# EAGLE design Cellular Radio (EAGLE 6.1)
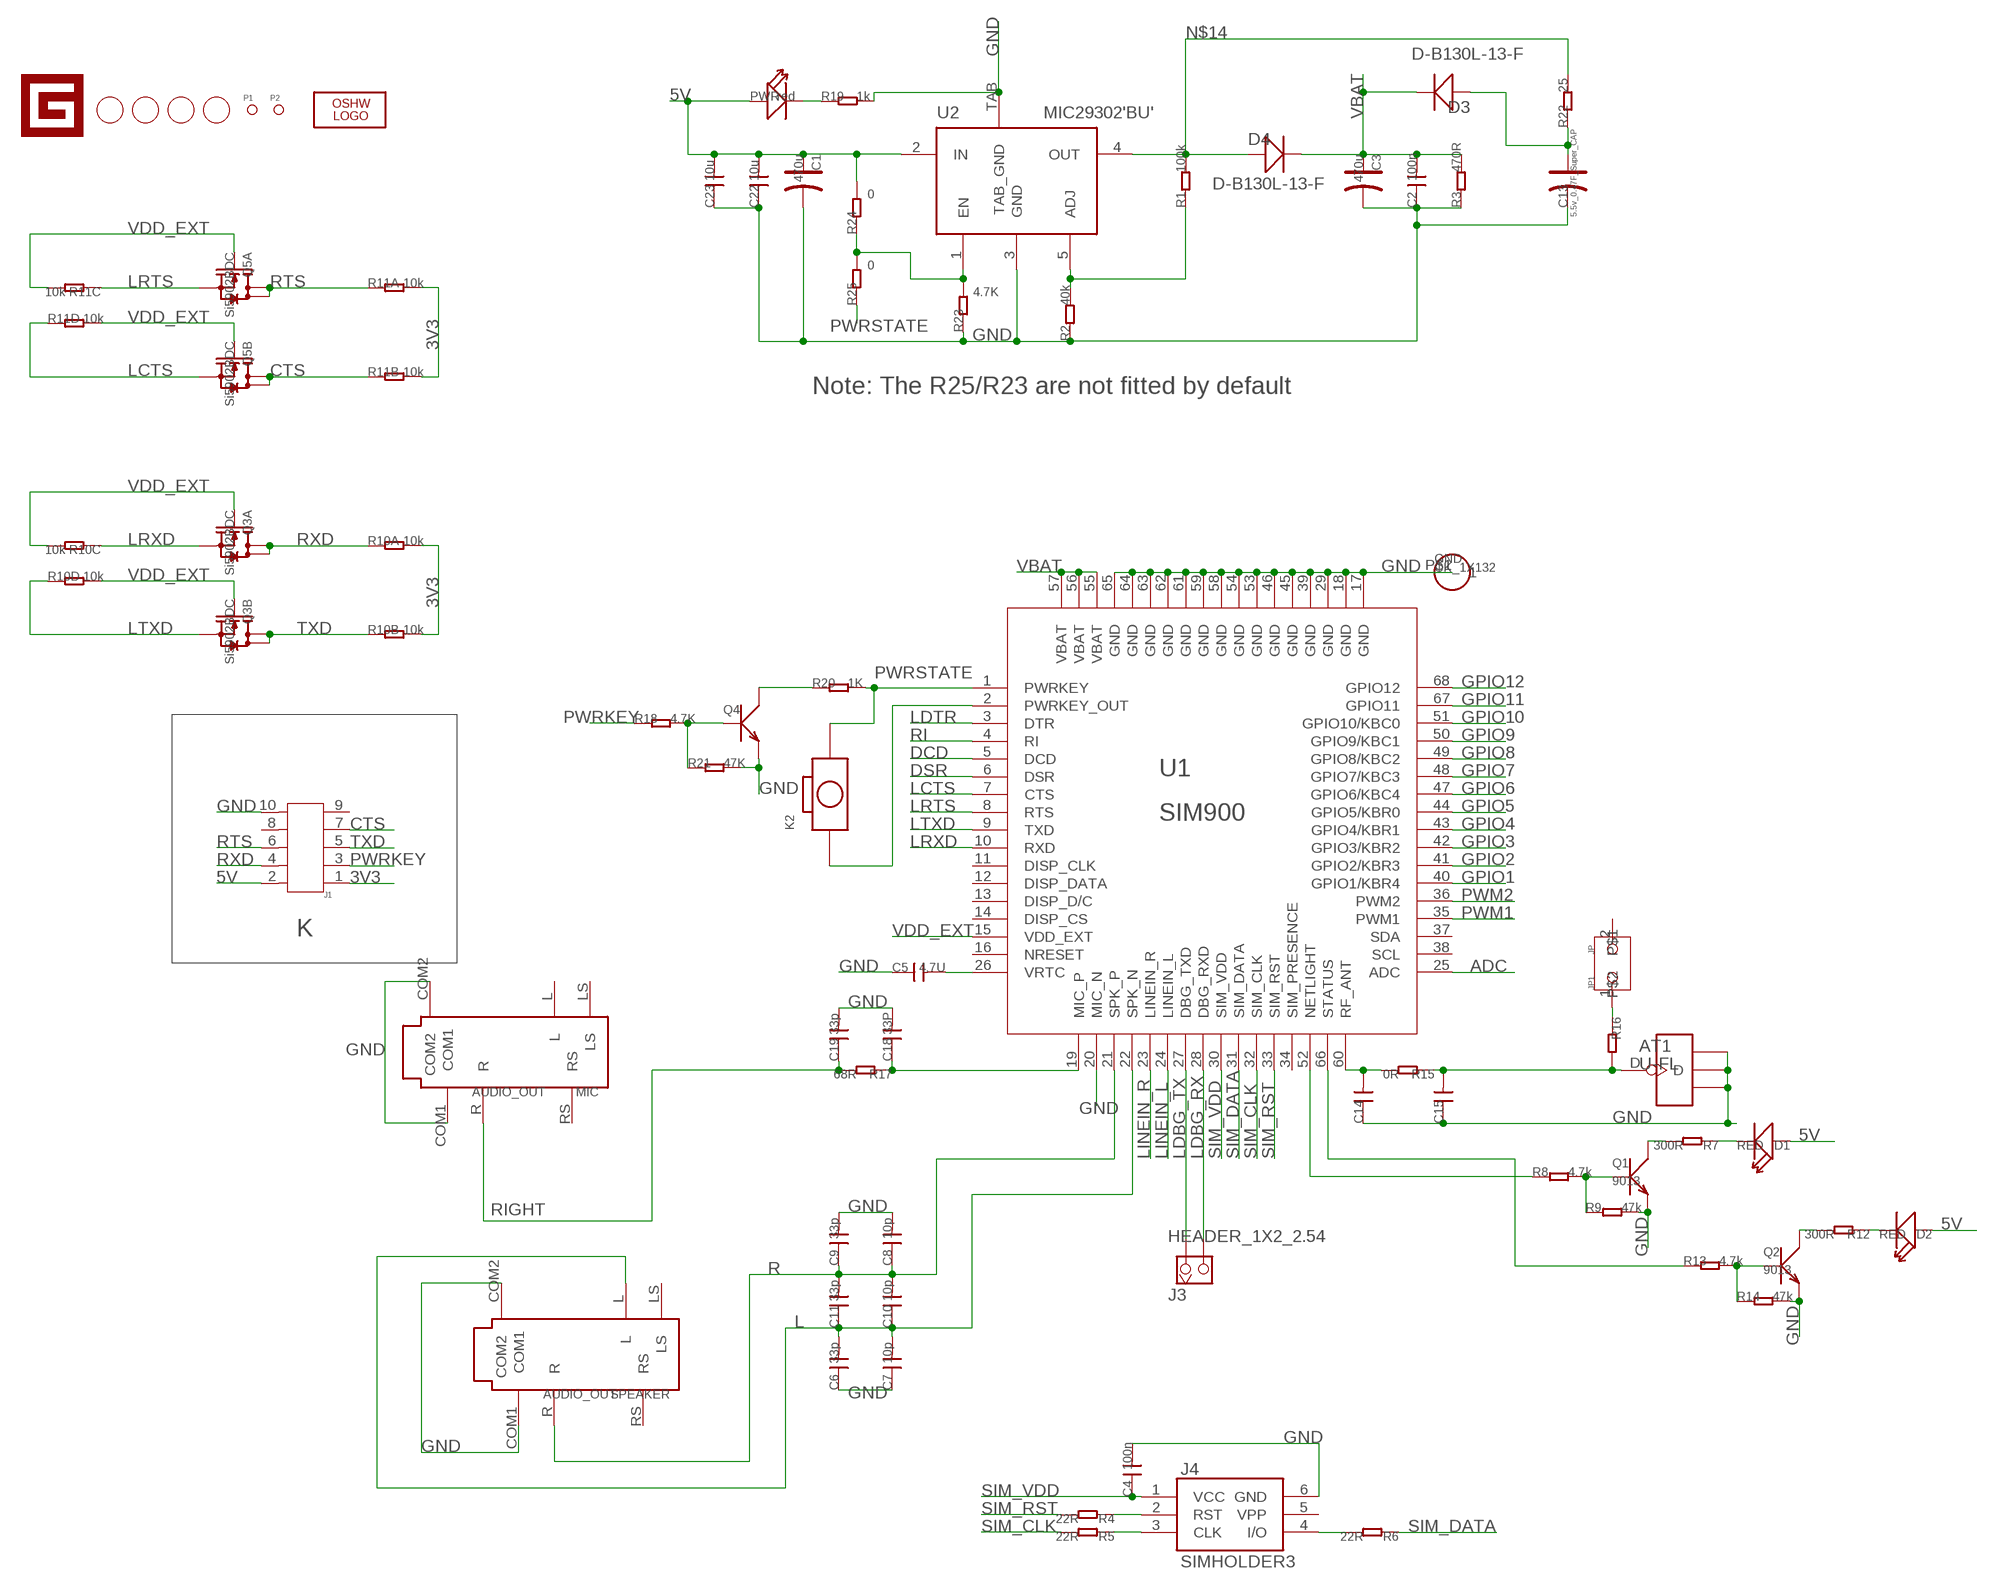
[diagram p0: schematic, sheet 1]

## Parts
AT1  U-FL  [U-FL]
C1  470u  006-CAP_AVX_D  [AVX_D]
C2  100n  006-C0805  [0805@1]
C3  470u  006-CAP_AVX_D  [AVX_D]
C4  100n  006-C0603  [0603@1]
C5  4.7U  006-C0805  [0805@1]
C6  33p  006-C0402  [0402]
C7  10p  006-C0402  [0402]
C8  10p  006-C0402  [0402]
C9  33p  006-C0402  [0402]
C10  10p  006-C0402  [0402]
C11  33p  006-C0402  [0402]
C13  5.5v_0.47F_Super_CAP  006-CAP_UC13  [SUPER_CAP_R13]
C14  006-C0402  [0402]
C15  006-C0402  [0402]
C18  33P  006-C0603  [0603@1]
C19  33p  006-C0603  [0603@1]
C22  10u  006-C0805  [0805@1]
C23  10u  006-C0805  [0805@1]
D1  RED  007-LED0603  [D0603]
D2  RED  007-LED0603  [D0603]
D3  D-B130L-13-F  [SMA]
D4  D-B130L-13-F  [SMA]
GND  CK_1X132  [CK_1X1]
J1  HEADER-SHF-105-01-L-D-SM  [SHF-105-01-L-D-SM]
J3  HEADER_1X2_2.54  [CK_1*2]
J4  SIMHOLDER3  [SIMHOLDER3]
JP1  JP  [JP]
K2  BOTTON_1_DP  [BTN_5.0_RST]
LOGO1  LOGO-OSHW-FILLX0150-NT  [OSHW_FILLX150_NOTEXT]
MIC  AUDIO_OUT  AUDIO  [3.5MM_AUDIO]
P1  PAD-MARK  [ROUND-MARK-0.635]
P2  PAD-MARK  [ROUND-MARK-0.635]
PWR  red  007-LED0603  [D0603]
Q1  9013  010-NPNSOT23  [SOT23]
Q2  9013  010-NPNSOT23  [SOT23]
Q3  Si5902BDC  010-DUAL-N-MOSFET_1206-8  [1206-8]
Q4  TRANSISTOR-NPN-SOT23''  [SOT23]
Q5  Si5902BDC  010-DUAL-N-MOSFET_1206-8  [1206-8]
R1  100k  005-R0805  [0805@1]
R2  40k  005-R0805  [0805@1]
R3  470R  005-R0805  [0805@1]
R4  22R  005-R0603  [0603@1]
R5  22R  005-R0603  [0603@1]
R6  22R  005-R0603  [0603@1]
R7  300R  005-R0603  [0603@1]
R8  4.7k  005-R0603  [0603@1]
R9  47k  005-R0603  [0603@1]
R10  10k  005-4R_1206  [R1206-8]
R11  10k  005-4R_1206  [R1206-8]
R12  300R  005-R0603  [0603@1]
R13  4.7k  005-R0603  [0603@1]
R14  47k  005-R0603  [0603@1]
R15  0R  005-R0402  [0402]
R16  005-R0402  [0402]
R17  68R  005-R0603  [0603@1]
R18  4.7K  005-R0402  [0402]
R19  1k  005-R0603  [0603@1]
R20  1K  005-R0402  [0402]
R21  47K  005-R0402  [0402]
R22  25  R-0603  [0603]
R23  4.7K  R-0603  [0603]
R24  0  R-0603  [0603]
R25  0  R-0603  [0603]
SPEAKER  AUDIO_OUT  AUDIO  [3.5MM_AUDIO]
U1  SIM900  [SIM900]
U2  MIC29302'BU'  [TO-263]
U$1  LOGO-GADGETEER-NORMAL  [GADGETEER-SILK]
U$2  PAD-HOLE'3.2/7.0'  [HOLE-D-3.2/7.0]
U$3  PAD-HOLE'3.2/7.0'  [HOLE-D-3.2/7.0]
U$4  PAD-HOLE'3.2/7.0'  [HOLE-D-3.2/7.0]
U$5  PAD-HOLE'3.2/7.0'  [HOLE-D-3.2/7.0]

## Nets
3V3: J1.1 R10.7 R10.8 R11.7 R11.8
5V: C1.+ C22.2 C23.2 D1.+ D2.+ J1.2 PWR.+ R24.2 U2.2(IN)
ADC: U1.25(ADC)
CTS: J1.7 Q5.5(B:D) Q5.6(B:D) R11.2
DCD: U1.5(DCD)
DSR: U1.6(DSR)
GND: AT1.GND1 AT1.GND2 AT1.GND3 C1.- C2.1 C3.- C4.2 C5.1 C6.1 C7.1 C8.2 C9.2 C13.- C14.1 C15.1 C18.2 C19.2 C22.1 C23.1 GND.P$1 J1.10 J4.6(GND) MIC.COM1 MIC.COM2 Q1.2(E) Q2.2(E) Q4.2(E) R2.1 R3.1 R9.2 R14.2 R19.2 R21.2 R23.1 SPEAKER.COM1 SPEAKER.COM2 U1.17(GND) U1.18(GND) U1.20(MIC_N) U1.29(GND) U1.39(GND) U1.45(GND) U1.46(GND) U1.53(GND) U1.54(GND) U1.58(GND) U1.59(GND) U1.61(GND) U1.62(GND) U1.63(GND) U1.64(GND) U1.65(GND) U2.3(GND) U2.TAB(TAB_GND)
GPIO1: U1.40(GPIO1/KBR4)
GPIO2: U1.41(GPIO2/KBR3)
GPIO3: U1.42(GPIO3/KBR2)
GPIO4: U1.43(GPIO4/KBR1)
GPIO5: U1.44(GPIO5/KBR0)
GPIO6: U1.47(GPIO6/KBC4)
GPIO7: U1.48(GPIO7/KBC3)
GPIO8: U1.49(GPIO8/KBC2)
GPIO9: U1.50(GPIO9/KBC1)
GPIO10: U1.51(GPIO10/KBC0)
GPIO11: U1.67(GPIO11)
GPIO12: U1.68(GPIO12)
L: C6.2 C7.2 C10.1 C11.1 SPEAKER.L U1.22(SPK_N)
LCTS: Q5.3(B:S) R11.4 U1.7(CTS)
LDBG_RX: J3.2 U1.28(DBG_RXD)
LDBG_TX: J3.1 U1.27(DBG_TXD)
LDTR: U1.3(DTR)
LINEIN_L: U1.24(LINEIN_L)
LINEIN_R: U1.23(LINEIN_R)
LRTS: Q5.1(A:S) R11.3 U1.8(RTS)
LRXD: Q3.1(A:S) R10.3 U1.10(RXD)
LTXD: Q3.3(B:S) R10.4 U1.9(TXD)
N$1: C14.2 R15.2 U1.60(RF_ANT)
N$2: R1.1 R2.2 U2.5(ADJ)
N$3: Q1.3(C) R7.2
N$4: J4.4(I/O) R6.2
N$5: J4.3(CLK) R5.1
N$6: J4.2(RST) R4.1
N$7: D1.- R7.1
N$8: Q1.1(B) R8.2 R9.1
N$9: Q4.3(C) R20.1
N$10: R8.1 U1.52(NETLIGHT)
N$11: Q4.1(B) R18.2 R21.1
N$12: C5.2 U1.26(VRTC)
N$13: C18.1 R17.1 U1.19(MIC_P)
N$14: D4.P$2(+) R1.2 R22.2 U2.4(OUT)
N$15: C13.+ D3.P$2(+) R22.1
N$16: Q2.3(C) R12.2
N$17: D2.- R12.1
N$18: Q2.1(B) R13.2 R14.1
N$19: R23.2 R24.1 R25.2 U2.1(EN)
N$20: R13.1 U1.66(STATUS)
N$21: AT1.D C15.2 R15.1 R16.2
N$22: JP1.1 R16.1
N$24: K2.P$1 U1.2(PWRKEY_OUT)
N$53: PWR.- R19.1
PWM1: U1.35(PWM1)
PWM2: U1.36(PWM2)
PWRKEY: J1.3 R18.1
PWRSTATE: K2.P$2 R20.2 R25.1 U1.1(PWRKEY)
R: C8.1 C9.1 C10.2 C11.2 SPEAKER.R U1.21(SPK_P)
RI: U1.4(RI)
RIGHT: C19.1 MIC.R R17.2
RTS: J1.6 Q5.7(A:D) Q5.8(A:D) R11.1
RXD: J1.4 Q3.7(A:D) Q3.8(A:D) R10.1
SIM_CLK: R5.2 U1.32(SIM_CLK)
SIM_DATA: R6.1 U1.31(SIM_DATA)
SIM_RST: R4.2 U1.33(SIM_RST)
SIM_VDD: C4.1 J4.1(VCC) U1.30(SIM_VDD)
TXD: J1.5 Q3.5(B:D) Q3.6(B:D) R10.2
VBAT: C2.2 C3.+ D3.P$1(-) D4.P$1(-) R3.2 U1.55(VBAT) U1.56(VBAT) U1.57(VBAT)
VDD_EXT: Q3.2(A:G) Q3.4(B:G) Q5.2(A:G) Q5.4(B:G) R10.5 R10.6 R11.5 R11.6 U1.15(VDD_EXT)
Unconnected: J1.8 J1.9 J4.5(VPP) JP1.2 MIC.L MIC.LS MIC.RS SPEAKER.LS SPEAKER.RS U1.11(DISP_CLK) U1.12(DISP_DATA) U1.13(DISP_D/C) U1.14(DISP_CS) U1.16(NRESET) U1.34(SIM_PRESENCE) U1.37(SDA) U1.38(SCL)

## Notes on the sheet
- Note: The R25/R23 are not fitted by default
- K

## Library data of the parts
AT1 = CPT_SMD:U-FL
C1 C3 C13 = Discrete:006-CAP*: Electrolytic Capacitors,Tantalum Capacitors and Super Capacitors
C2 C4-C11 C14 C15 C18 C19 C22 C23 = Discrete:006-C*: Ceramic Capacitors
D1 D2 PWR = Discrete:007-LED*
D3 D4 = Discrete:D*
GND = CONNECTER:CK_1X1
J1 = Connector:HEADER-SHF-105-01-L-D-SM
J3 = CONNECTER:HEADER_1X2
J4 = SparkFun2:SIMHOLDER3
JP1 = mySeeed:JP
K2 = CPT_SMD:BOTTON_1
LOGO1 = Logo:LOGO-OSHW-FILL
MIC SPEAKER = MusicShield:AUDIO
P1 P2 = Discreter:PAD-MARK
Q1 Q2 = Discrete:010-NPN*: NPN audion
Q3 Q5 = Discrete:010-DUAL-N-MOSFET*: Si5902BDC Si5904DC Si5908DC Si5920DC
Q4 = Discreter:TRANSISTOR-NPN*: NPN audion
R1-R9 R12-R21 = Discrete:005-R*
R10 R11 = Discrete:005-4R*: Resistor Array
R22-R25 = Discrete:R*
U1 = ICs_v54:SIM900
U2 = ICs_v54:MIC29302
U$1 = Logo:LOGO-GADGETEER
U$2-U$5 = Discreter:PAD-HOLE

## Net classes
0 default: width 0.203 mm, drill 0.305 mm, clearance 0.152 mm

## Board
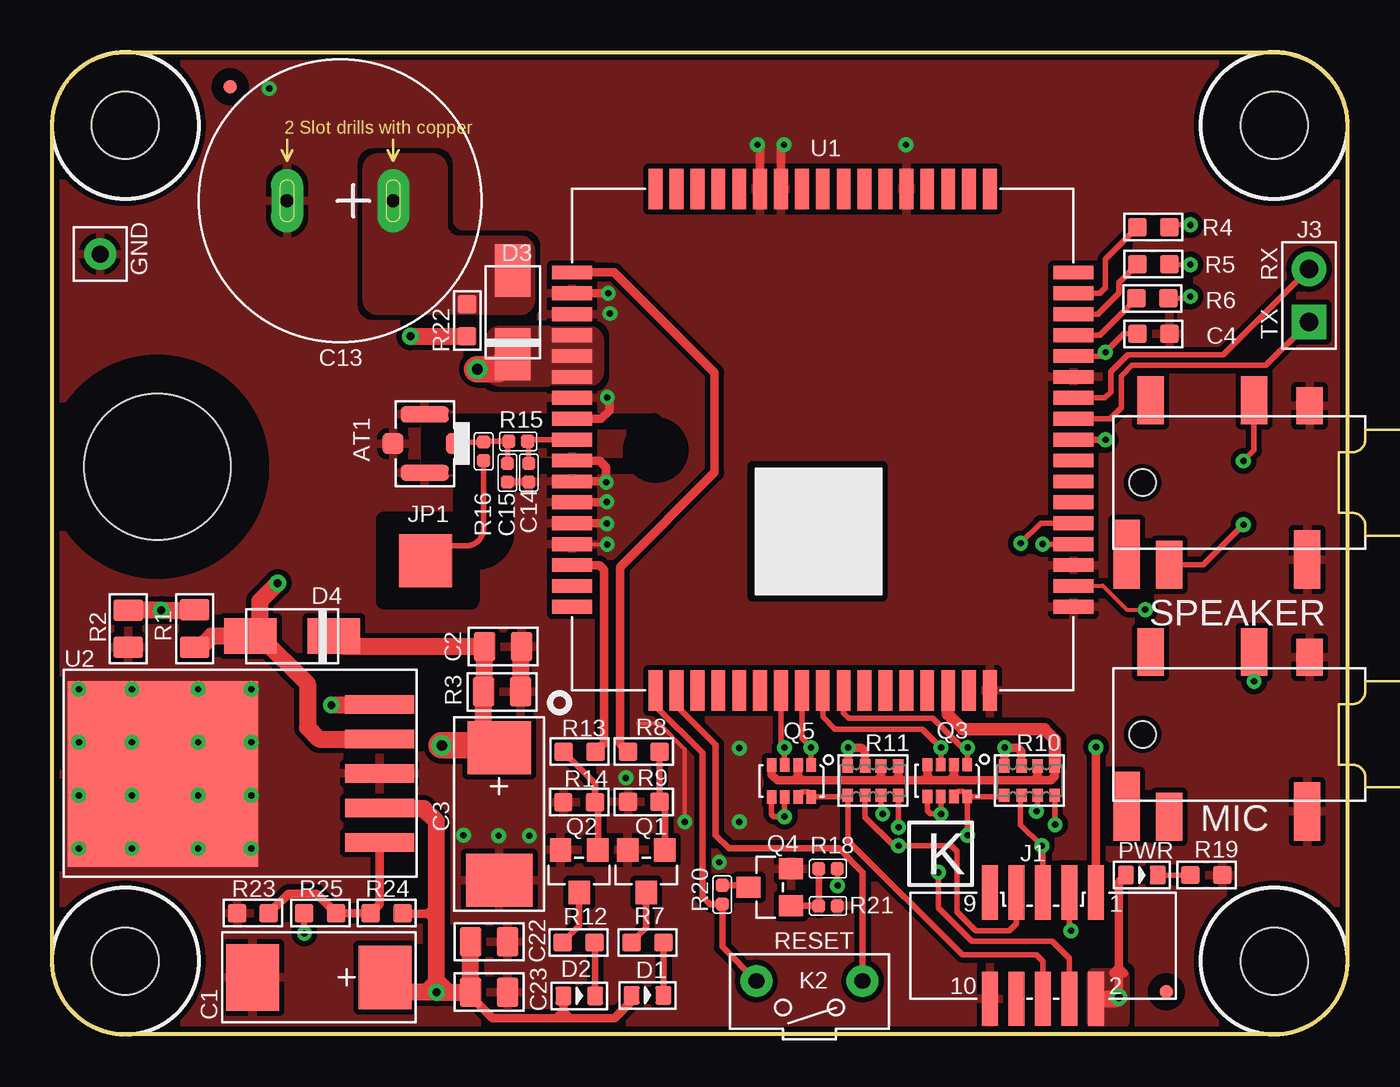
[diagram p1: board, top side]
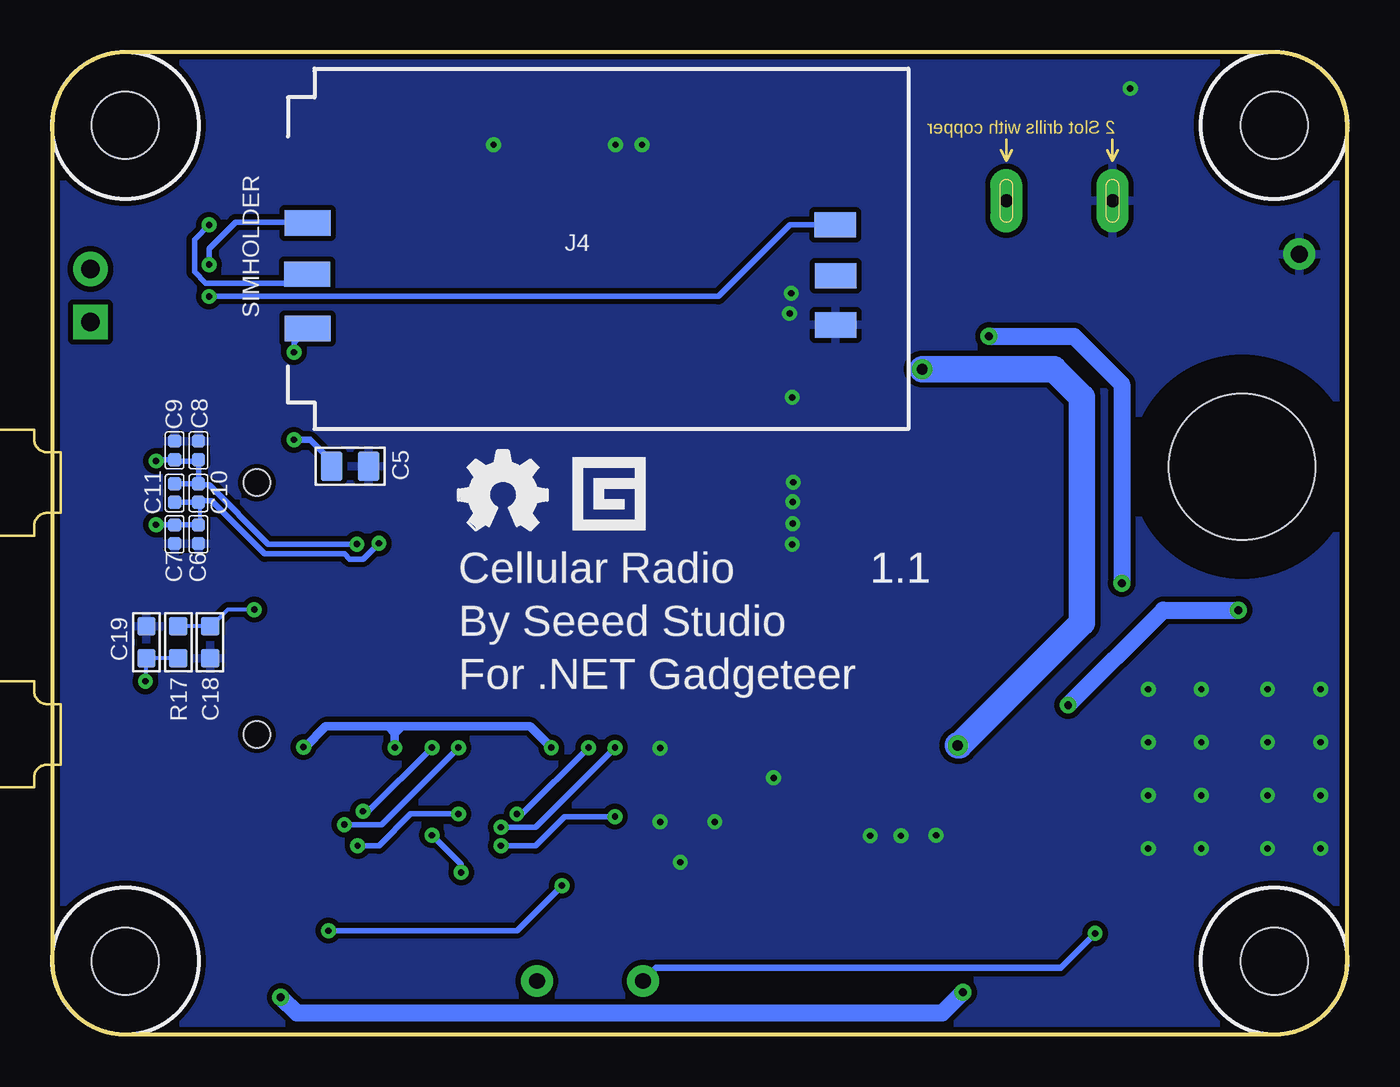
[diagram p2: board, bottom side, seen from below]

Size 62 x 47 mm. Coordinates in mm from the lower left corner, seen from the top.
Outline: 62,3.5 arc-90 58.5,0 3.5,0 arc-90 0,3.5 0,43.5 arc-90 3.5,47 58.5,47 arc-90 62,43.5 62,3.5
Copper layers (1*16): Top 0.035mm / dielectric 1.5mm / Bottom 0.035mm
Design rules: minimum track width 8mil, minimum drill 12mil, track to track 6mil, track to pad 6mil, pad to pad 6mil, via to via 6mil, smd to smd 6mil, copper to edge 10mil, drill to drill 8mil, minimum pad ring 10mil, minimum via ring 8mil, stop-mask expansion 4mil, vias tented up to drill 100mil, thermal gap 10mil
Holes 7 mm at 5.04,27.16
tRestrict: area 0,22.2 to 10,32.2; area 24.1,34.8 to 25.5,35.2; area 24.3,29.7 to 25.7,30.1; area 24.1,23.8 to 25.5,24.1; area 24.1,25.8 to 25.5,26.2; area 24.1,24.8 to 25.5,25.2; area 34.2,39.8 to 34.5,41.2; area 33.5,21 to 39.8,27.2; 14 lines
bRestrict: area 0,22.2 to 10,32.2

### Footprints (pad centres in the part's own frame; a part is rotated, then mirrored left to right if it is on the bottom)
U-FL = smd 1.016 x 1.016: D -1.524,0; GND3 1.524,0 | smd 2.286 x 0.762: GND1 0,1.397; GND2 0,-1.397
AVX_D = smd 2.54 x 3.048: + -3.175,0 | smd 2.54 x 3.175: - 3.175,0
0805@1 = smd 1.016 x 1.397: 1 -0.889,0; 2 0.889,0
0603@1 = smd 0.889 x 0.889: 1 -0.762,0; 2 0.762,0
0402 = smd 0.635 x 0.635: 1 -0.445,0; 2 0.445,0
SUPER_CAP_R13 = drill 0.635 pad 1.524 long: + -2.54,0; - 2.54,0
D0603 = smd 0.762 x 0.889: + -0.762,0; - 0.762,0
SMA = smd 2.5 x 1.7: P$1 -2,0; P$2 2,0
CK_1X1 = drill 0.813 pad 1.524: P$1 0,0
SHF-105-01-L-D-SM = smd 0.762 x 2.6: 1 -2.54,-2.54; 2 -2.54,2.54; 3 -1.27,-2.54; 4 -1.27,2.54; 5 0,-2.54; 6 0,2.54; 7 1.27,-2.54; 8 1.27,2.54; 9 2.54,-2.546; 10 2.54,2.54
CK_1*2 = drill 0.889 pad 1.651 square: 1 0,1.27 | drill 0.889 pad 1.651: 2 0,-1.27
SIMHOLDER3 = smd 2.2 x 1.2: 1 0.95,4.81; 2 0.91,7.41; 3 0.95,9.86 | smd 2 x 1.2: 4 26.2,9.78; 5 26.22,7.34; 6 26.22,4.98
JP = smd 1.27 x 2.54: 1 -0.635,0; 2 0.635,0
BTN_5.0_RST = drill 0.762 pad 1.524: P$1 0,2.54; P$2 0,-2.54
3.5MM_AUDIO = smd 1.27 x 1.778: COM1 -4.572,3.683 | smd 1.27 x 2.794: COM2 -4.699,-3.683 | smd 1.27 x 2.286: L -11.303,-3.937; R -7.239,3.937; RS -12.192,3.937 | smd 1.27 x 3.302: LS -13.335,-3.429 | hole 1.27: -12.573,0
ROUND-MARK-0.635 = smd 0.635 x 0.635: P$1 0,0
SOT23@1 = smd 1.016 x 1.143: 1 -0.889,-1.016; 2 0.889,-1.016; 3 0,1.016
1206-8 = smd 0.457 x 0.635: 1 -0.953,-0.762; 2 -0.318,-0.762; 3 0.318,-0.762; 4 0.953,-0.762; 5 0.953,0.762; 6 0.318,0.762; 7 -0.318,0.762; 8 -0.953,0.762
SOT23 = smd 1.016 x 1.143: 1 -0.889,-1.016; 2 0.889,-1.016; 3 0,1.016
R1206-8 = smd 0.508 x 0.635: 1 -1.206,-0.699; 2 -0.381,-0.699; 3 0.381,-0.699; 4 1.206,-0.699; 5 1.206,0.699; 6 0.381,0.699; 7 -0.381,0.699; 8 -1.206,0.699
0603 = smd 0.889 x 0.889: 1 -0.762,0; 2 0.762,0
SIM900 = smd 1.93 x 0.66: 1 -12,8; 2 -12,7; 3 -12,6; 4 -12,5; 5 -12,4; 6 -12,3; 7 -12,2; 8 -12,1; 9 -12,0; 10 -12,-1; 11 -12,-2; 12 -12,-3; 13 -12,-4; 14 -12,-5; 15 -12,-6; 16 -12,-7; 17 -12,-8; 35 12,-8; 36 12,-7; 37 12,-6; 38 12,-5; 39 12,-4; 40 12,-3; 41 12,-2; 42 12,-1; 43 12,0; 44 12,1; 45 12,2; 46 12,3; 47 12,4; 48 12,5; 49 12,6; 50 12,7; 51 12,8 | smd 0.66 x 1.93: 18 -8,-12; 19 -7,-12; 20 -6,-12; 21 -5,-12; 22 -4,-12; 23 -3,-12; 24 -2,-12; 25 -1,-12; 26 0,-12; 27 1,-12; 28 2,-12; 29 3,-12; 30 4,-12; 31 5,-12; 32 6,-12; 33 7,-12; 34 8,-12; 52 8,12; 53 7,12; 54 6,12; 55 5,12; 56 4,12; 57 3,12; 58 2,12; 59 1,12; 60 0,12; 61 -1,12; 62 -2,12; 63 -3,12; 64 -4,12; 65 -5,12; 66 -6,12; 67 -7,12; 68 -8,12
TO-263 = smd 3.302 x 0.889: 1 3.302,-3.302; 2 3.302,-1.651; 3 3.302,0; 4 3.302,1.651; 5 3.302,3.302 | smd 9.12 x 8.89: TAB -7.071,-0.03
HOLE-D-3.2/7.0 = hole 3.2: 0,0

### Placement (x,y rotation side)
AT1  17.83,28.27 180 top
C1  12.76,2.73 180 top
C2  21.59,18.56 180 top
C3  21.4,10.54 270 top
C4  52.72,33.53 0 top
C5  47.74,27.19 180 bottom
C6  55,23.93 90 bottom
C7  56.14,23.93 90 bottom
C8  55,27.95 90 bottom
C9  56.14,27.95 90 bottom
C10  55,25.91 90 bottom
C11  56.14,25.91 90 bottom
C13  13.78,39.89 180 top
C14  22.81,26.88 90 top
C15  21.8,26.88 90 top
C18  54.44,18.76 270 bottom
C19  57.49,18.76 90 bottom
C22  20.92,4.44 180 top
C23  20.92,2.02 180 top
D1  28.5,1.86 0 top
D2  25.23,1.84 0 top
D3  22.05,34.55 90 top
D4  11.49,19.05 180 top
GND  2.29,37.34 0 top
J1  47.43,4.24 180 top
J3  60.17,35.36 180 top
J4  50.71,28.97 0 bottom
JP1  17.87,22.66 270 top
K2  36.25,2.55 270 top
LOGO1  42.55,24.14 0 bottom
MIC  64.78,14.36 0 top
P1  8.51,45.34 0 top
P2  53.34,2.04 0 top
PWR  52.16,7.62 0 top
Q1  9013  [SOT23@1]  28.44,7.81 180 top
Q2  9013  [SOT23@1]  25.23,7.81 180 top
Q3  42.85,12.14 180 top
Q4  34.35,7.04 90 top
Q5  35.39,12.12 180 top
R1  6.82,19.42 270 top
R2  3.64,19.41 90 top
R3  21.54,16.39 180 top
R4  52.72,38.63 180 top
R5  52.72,36.86 180 top
R6  52.67,35.22 0 top
R7  28.5,4.4 180 top
R8  28.32,13.53 0 top
R9  28.32,11.13 180 top
R10  46.79,12.14 0 top
R11  39.3,12.14 0 top
R12  25.2,4.4 180 top
R13  25.25,13.53 180 top
R14  25.23,11.11 180 top
R15  22.31,28.38 0 top
R16  20.65,27.9 90 top
R17  55.97,18.76 270 bottom
R18  37.14,7.93 180 top
R19  55.26,7.62 0 top
R20  32.08,6.69 270 top
R21  37.14,6.15 0 top
R22  19.87,34.17 270 top
R23  9.61,5.8 0 top
R24  16.01,5.8 0 top
R25  12.83,5.8 0 top
SPEAKER  64.78,26.41 0 top
U1  36.89,28.46 90 top
U2  12.37,12.49 0 top
U$1  34.93,26.29 0 bottom
U$2  3.5,3.5 0 top
U$3  3.5,43.5 0 top
U$4  58.5,43.5 0 top
U$5  58.5,3.5 0 top

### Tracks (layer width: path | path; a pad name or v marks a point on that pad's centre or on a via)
3V3  (via drill 0.3 pad 0.64)
  Top 0.406: R11.8 38.09,13.7 v38.11,13.72 38.74,13.72 38.91,13.55 R11.7 | R10.8 45.58,13.7 v45.6,13.72 46.23,13.72 46.41,13.55 R10.7 | J1.1 v49.97,13.74 v49.97,13.75
  Bottom 0.406: v38.11,13.72 39.12,14.74 45.27,14.74 | 45.6,14.74 45.93,14.74 | v49.97,13.75 49.89,13.75 48.9,14.74 45.93,14.74 | 45.6,14.41 45.6,14.74 | v45.6,13.72 45.6,14.25 45.6,14.41 | 45.27,14.74 45.6,14.41 | 45.27,14.74 45.6,14.74 | 45.6,14.41 45.93,14.74
5V  (via drill 0.38 pad 0.81)
  Top 0.254: 17.96,5.8 17.96,5.77
  Top 0.305: 27.74,1.7 D1.+
  Top 0.406: 27.74,1.7 27.74,1.58 26.93,0.77 24.77,0.77 | 24.14,0.77 24.39,0.77 | 24.39,0.77 24.77,0.77 | 24.47,1.07 24.47,0.85 24.39,0.77 | 24.47,1.1 D2.+ | 24.14,0.77 24.47,1.1 | 24.47,1.1 24.47,1.07 | 24.47,1.07 24.77,0.77 | 24.14,0.77 21.09,0.77 20.08,1.77 20.08,1.97 | 18.39,5.85 18.34,5.8 17.96,5.8 18.42,5.34 | 18.42,6.23 17.96,5.77 16.79,5.77 R24.2 | 16.52,10.8 15.67,10.8 U2.2 | v51.06,1.78 51.06,3.18 | 51.06,3.18 51.06,7.28 PWR.+ | 51.06,3.18 50.8,2.93 | 51.06,3.18 51.31,2.93
  Top 0.813: J1.2 50.98,1.7 v51.06,1.78 | 15.71,10.8 16.52,10.8 17.79,10.8 18.39,10.19 18.39,5.85 18.39,2.7 | v18.39,2.01 C23.2 | 18.42,2.55 18.4,2.57 18.4,2.69 18.39,2.7 | 18.42,2.55 18.93,2.04 | 18.42,2.55 17.89,2.02 | v18.39,2.01 16.65,2.01 C1.+ | v18.39,2.01 18.39,2.7 | C23.2 C22.2 | C23.2 arc-60 20.08,1.97
  Bottom 0.813: v51.06,1.78 50.3,1.02 19.38,1.02 v18.39,2.01
  pour Top (isolate 0.254, no thermals): 51.44,0.64 arc-90 51.19,0.39 49.92,0.39 arc-90 49.66,0.64 49.66,2.8 arc-90 49.92,3.05 51.19,3.05 arc-90 51.44,2.8
CTS  (via drill 0.3 pad 0.64)
  Top 0.254: Q5.6 35.06,11.35 v35.06,10.42 34.55,10.42 34.44,10.53 Q5.5 | J1.7 46.16,5.3 45.82,4.96 44.23,4.96 43.31,5.87 43.31,8.77 43.06,9.02 v40.52,9.02 40.29,9.02 38.91,10.4 R11.2
  Bottom 0.254: v35.06,10.42 37.47,10.42 38.87,9.02 v40.52,9.02
GND  (via drill 0.3 pad 0.64)
  Top 0.203: v30.28,10.16 30.28,13.64 29.06,14.86 28.05,14.86 | U1.65 v26.56,23.46 v26.57,23.45
  Top 0.305: C15.1 C14.1
  Top 0.406: U1.61 26.2,27.46 26.52,27.13 26.52,26.68 | 26.52,26.68 v26.52,26.42 | U1.62 26.31,26.46 26.52,26.68 | U1.63 26.53,25.46 v26.55,25.48 | U1.64 26.57,24.46 v26.55,24.44 | U1.46 33.89,42.45 v33.76,42.58 | U1.45 34.89,42.43 v35.03,42.58 | U1.53 v26.62,35.46 | U1.59 26.29,29.46 26.68,29.85 26.68,30.38 v26.57,30.48
  Top 0.813: R3.1 22.43,18.51 C2.1
  other vias: 32.9,10.16 1.27,16.52 3.82,16.52 6.99,16.52 9.53,16.52 1.27,13.97 1.27,11.44 1.27,8.89 3.82,13.97 6.99,13.97 9.53,13.97 9.53,11.44 9.53,8.89 6.99,8.89 3.82,8.89 3.82,11.44 6.99,11.44 32.9,13.7 27.46,12.27 19.69,9.53 22.84,9.5 21.37,9.5 31.93,8.23 40.87,42.58 26.7,34.5 10.39,45.27
  pour Bottom (isolate 0.254, rank 5): -0.23,47 62.23,47 62.23,-0.63 -0.23,-0.63
  pour Top (isolate 0.254, rank 5): -0.23,47 62.23,47 62.23,-0.63 -0.23,-0.63
  pour Top (isolate 0.254, no thermals): 0.64,17.15 10.8,17.15 10.8,7.62 0.64,7.62
L  (via drill 0.3 pad 0.64)
  Top 0.254: U1.22 47.32,24.46 v46.36,23.5 | SPEAKER.L 55.11,22.47 v57.03,24.39
  Bottom 0.203: C10.1 54.94,25.41 54.94,24.43 C6.2
  Bottom 0.254: v46.36,23.5 47.12,22.74 47.76,22.74 48.01,22.99 51.82,22.99 54.36,25.53 54.92,25.53 C10.1 | C10.1 C11.1 | C10.1 55.01,25.45 | C6.2 C7.2 56.16,24.39 v57.03,24.39
LCTS  (via drill 0.3 pad 0.64)
  Top 0.254: Q5.3 35.06,12.9 v35.06,13.72 34.89,13.89 U1.7 | R11.4 40.5,9.93 v40.52,9.91
  Bottom 0.254: v40.52,9.91 38.87,9.91 v35.06,13.72
LDBG_RX
  Top 0.254: U1.28 50.4,30.46 50.68,30.74 50.68,31.7 51.49,32.52 56.06,32.52 J3.2
LDBG_TX
  Top 0.254: U1.27 50.67,29.46 51.19,29.98 51.19,31.5 51.69,32.01 58.09,32.01 J3.1
LRTS  (via drill 0.3 pad 0.64)
  Top 0.254: R11.3 39.68,10.63 v39.76,10.55 | Q5.1 36.33,12.9 v36.33,13.72 35.89,14.16 U1.8
  Bottom 0.254: v39.76,10.55 39.5,10.55 v36.33,13.72
LRXD  (via drill 0.3 pad 0.64)
  Top 0.254: R10.3 47.17,10.72 v47.12,10.67 | Q3.1 43.82,12.92 v43.82,13.72 43.57,13.72 42.17,15.12 38.14,15.12 37.89,15.37 U1.10
  Bottom 0.254: v47.12,10.67 46.87,10.67 v43.82,13.72
LTXD  (via drill 0.3 pad 0.64)
  Top 0.254: R10.4 47.99,10.05 v48.01,10.04 | Q3.3 42.55,12.92 v42.55,13.72 41.66,14.61 37.47,14.61 36.89,15.19 U1.9
  Bottom 0.254: v48.01,10.04 46.23,10.04 v42.55,13.72
N$1
  Top 0.254: U1.60 22.75,28.46 R15.2 22.81,28.38 C14.2
N$2  (via drill 0.38, 0.38 pad 0.81)
  Top 0.813: v13.37,15.75 15.64,15.75 U2.5 | v5.21,20.3 6.79,20.3 arc45 R1.1 6.81,20.3 v5.21,20.3 | v5.21,20.3 R2.2
  Bottom 0.813: v13.37,15.75 8.82,20.3 v5.21,20.3
N$3
  Top 0.305: Q1.3 28.44,5.1 R7.2
N$4  (via drill 0.3 pad 0.64)
  Top 0.254: R6.2 54.4,35.22 v54.49,35.31
  Bottom 0.254: v54.49,35.31 30.1,35.31 26.68,38.74 J4.4
N$5  (via drill 0.3 pad 0.64)
  Top 0.254: v54.49,36.84 53.5,36.84 R5.1
  Bottom 0.254: v54.49,36.84 54.49,37.6 53.22,38.87 49.8,38.87 J4.3
N$6  (via drill 0.3 pad 0.64)
  Top 0.254: v54.49,38.74 53.59,38.74 R4.1
  Bottom 0.254: J4.2 50.37,36.38 50.8,35.95 54.65,35.95 55.19,36.48 55.19,38.04 v54.49,38.74
N$7
  Top 0.305: R7.1 D1.-
N$8
  Top 0.305: Q1.1 29.33,10.88 R9.1 R8.2
N$9
  Top 0.305: R20.1 33.24,7.13 Q4.3
N$10
  Top 0.406: U1.52 26.93,36.46 31.71,31.67 31.71,26.89 27.18,22.36 27.18,13.9 R8.1
N$11
  Top 0.305: Q4.1 R21.1 R18.2
N$12  (via drill 0.3 pad 0.64)
  Top 0.305: v50.42,28.45 U1.26
  Bottom 0.305: C5.2 48.62,27.42 49.66,28.45 v50.42,28.45
N$13  (via drill 0.3 pad 0.64)
  Top 0.203: U1.19 50.3,21.47 51.44,20.32 v52.33,20.32
  Bottom 0.203: R17.1 C18.1 54.4,19.52 53.6,20.32 v52.33,20.32
N$14  (via drill 0.38 pad 0.81)
  Top 0.813: 9.94,19.05 D4.P$2 7.62,19.05 7.12,18.55 6.83,18.55 R1.2 | 9.94,19.05 12.22,16.77 12.22,14.69 12.78,14.13 15.66,14.13 U2.4 | 9.94,19.05 9.94,20.73 v10.8,21.59 | v17.15,33.41 R22.2
  Bottom 0.813: v10.8,21.59 10.8,31.12 13.09,33.41 v17.15,33.41
N$15
  pour Top (isolate 0.254, no thermals): 22.36,34.55 arc90 22.99,35.18 22.99,37.47 arc90 22.36,38.11 19.44,38.11 arc-90 18.8,38.74 18.8,41.41 arc90 18.17,42.04 15.63,42.04 arc90 14.99,41.41 14.99,35.18 arc90 15.63,34.55
N$16
  Top 0.305: Q2.3 25.23,5.19 R12.2
N$17
  Top 0.305: D2.- 25.99,4.36 R12.1
N$18
  Top 0.305: Q2.1 26.12,10.98 R14.1 25.99,12.02 R13.2
N$19
  Top 0.406: R23.2 11.31,6.74 12.65,6.74 R25.2 R24.1 15.67,6.22 U2.1
N$20
  Top 0.406: U1.66 26.19,22.46 26.42,22.23 26.42,14.48 26.42,13.94 R13.1
N$21
  Top 0.254: 21.8,28.38 R15.1 | 21.8,28.38 C15.2 | 21.8,28.38 20.69,28.38 R16.2 19.43,28.34 AT1.D
N$22
  Top 0.254: R16.1 20.65,24.23 arc-90 19.79,23.37 17.95,23.37 JP1.1
N$24
  Top 0.305: U1.2 29.89,15.71 31.76,13.85 31.76,9.53 32.39,8.89 37.66,8.89 38.79,7.76 K2.P$1
N$53
  Top 0.254: PWR.- R19.1
PWRKEY  (via drill 0.3 pad 0.64)
  Top 0.254: J1.3 48.7,5.03 v48.77,4.96 | v37.6,7.12 37.6,7.92 R18.1
  Bottom 0.254: v48.77,4.96 39.76,4.96 v37.6,7.12
PWRSTATE  (via drill 0.3 pad 0.64)
  Top 0.305: U1.1 28.89,15.7 31.12,13.47 31.12,6.61 31.5,6.23 32.07,6.23 R20.2 32.08,4.18 K2.P$2 | v12.07,4.83 R25.1
  Bottom 0.305: K2.P$2 33.09,3.18 14.1,3.18 13.97,3.18 13.72,3.18 v12.07,4.83
R  (via drill 0.3 pad 0.64)
  Top 0.254: U1.21 v47.42,23.46 47.38,23.5 | SPEAKER.R 57.54,27.95 v57.03,27.44
  Bottom 0.254: v47.42,23.46 51.65,23.46 54.49,26.29 54.94,26.29 C10.2 | C10.2 C11.2 | C10.2 55,27.44 | 55,27.44 C8.1 | 55,27.44 56.08,27.44 C9.1 56.97,27.5 v57.03,27.44
RIGHT  (via drill 0.3 pad 0.64)
  Top 0.203: v57.54,16.9 MIC.R
  Bottom 0.203: v57.54,16.9 57.54,17.95 C19.1 R17.2
RTS
  Top 0.254: J1.6 47.43,3.5 47.12,3.82 43.57,3.82 38.11,9.28 38.11,11.43 R11.1 38.01,11.36 Q5.8 36.34,11.42 36.16,11.61 35.92,11.61 35.71,11.4 Q5.7
RXD  (via drill 0.3 pad 0.64)
  Top 0.254: Q3.7 43.17,11.42 43.38,11.63 43.59,11.63 43.8,11.42 Q3.8 | Q3.8 45.52,11.38 R10.1 | J1.4 48.7,3.63 47.88,4.45 44.03,4.45 42.42,6.06 v42.42,7.75 | v43.82,9.53 43.82,11.36 Q3.8
  Bottom 0.254: v42.42,7.75 42.42,8.13 v43.82,9.53
SIM_CLK
  Top 0.254: U1.32 50.05,34.46 51.06,35.47 51.06,35.96 R5.2
SIM_DATA
  Top 0.254: U1.31 50.14,33.46 51.44,34.76 R6.1
SIM_RST
  Top 0.254: U1.33 50.16,35.46 50.42,35.73 50.42,37.1 R4.2
SIM_VDD  (via drill 0.3 pad 0.64)
  Top 0.254: U1.30 50.24,32.46 v50.42,32.64 51.31,33.53 C4.1
  Bottom 0.254: v50.42,32.64 50.42,33.12 J4.1
TXD  (via drill 0.3 pad 0.64)
  Top 0.254: R10.2 46.36,11.4 46.36,10.04 v47.38,9.02 47.43,8.97 J1.5 | Q3.6 42.55,11.36 v42.55,10.55 42.04,10.55 41.9,10.69 Q3.5
  Bottom 0.254: v42.55,10.55 44.84,10.55 46.36,9.02 v47.38,9.02
VBAT  (via drill 0.51 pad 0.97)
  Top 0.813: C3.+ 20.65,14.46 R3.2 20.7,16.43 C2.2 13.98,18.56 D4.P$1
  Top 1.27: v20.35,31.83 21.33,31.83 D3.P$1 | v18.65,13.82 21.29,13.82 C3.+
  Bottom 1.27: v18.65,13.82 18.57,13.82 12.71,19.69 12.71,30.48 14.05,31.83 v20.35,31.83
  pour Top (isolate 0.254, no thermals): 20.83,33.15 arc-90 21.47,33.79 25.66,33.79 arc-90 26.29,33.15 26.29,31.76 arc-90 25.66,31.12 21.47,31.12 arc-90 20.83,31.76
VDD_EXT
  Top 0.203: 36.05,12.17 35.71,12.17 35.71,12.47 35.72,12.48 35.67,12.48 35.36,12.17 | 36.05,12.17 36.07,12.2 | 47.17,12.37 47.17,12.4 47.12,12.45 | 47.17,12.23 47.17,12.37 | 47.17,12.37 47.25,12.45 | 43.17,12.17 43.41,12.17 43.44,12.2 | 43.44,12.2 43.69,12.2 | 41.9,12.56 41.9,12.69 | 41.9,12.69 41.91,12.71 41.91,12.58 41.9,12.56 | 41.9,12.17 41.9,12.51 | 39.68,12.37 39.68,12.4 39.63,12.45 39.32,12.15 | 39.68,12.23 39.68,12.37 | 39.68,12.37 39.76,12.45 | 36.05,12.17 35.74,12.48 | 40.85,12.15 40.54,12.45 40.52,12.45 | 43.44,12.25 43.54,12.15 | 47.55,12.1 47.25,12.4 47.25,12.76 R10.6 | 46.74,12.07 47.05,12.38 47.05,12.21 47,12.15 | 43.13,12.5 42.83,12.2 43.14,12.2 43.19,12.15 | R11.6 39.76,12.76 39.76,12.43 40.06,12.12 40.14,12.12 40.47,12.45 40.52,12.45 | 40.5,12.43 40.52,12.45 | 41.9,12.56 41.9,12.51 | 41.9,12.51 41.86,12.48 | 41.86,12.48 41.56,12.17 | 41.86,12.48 41.94,12.48 42.27,12.15 | 41.86,12.48 41.86,12.65 41.9,12.69 | 43.44,12.2 43.44,12.25 | 43.44,12.25 43.24,12.45
  Top 0.406: Q5.4 34.44,12.43 34.72,12.15 35.69,12.15 35.71,12.17 | 39.76,12.15 40.39,12.15 | 40.39,12.15 41.91,12.15 | 41.91,12.15 43.19,12.15 | 43.19,12.15 47,12.15 47.25,12.15 | 47.25,12.15 47.81,12.15 48.01,12.35 48.01,12.82 R10.5 | R10.6 47.17,12.23 47.25,12.15 | Q3.2 43.17,12.17 43.19,12.15 | Q3.4 41.9,12.56 41.9,12.17 41.91,12.15 | R11.5 40.5,12.43 40.5,12.27 40.39,12.15 | R11.6 39.68,12.23 39.76,12.15 | 35.71,12.17 Q5.2 | 39.76,12.15 35.73,12.15 35.71,12.17
  Top 0.61: U1.15 42.89,15.32 43.6,14.61 47.5,14.61 48.01,14.1 48.01,12.86 R10.5

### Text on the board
tPlace: RX | TX | K | RESET | C22
bPlace: SIMHOLDER | 1.1 | Cellular Radio | By Seeed Studio | For .NET Gadgeteer
bNames: J4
